|   IBIS model for TI am5k2e04 DSP
| -This IBIS model also supports am5k2e02
[IBIS Ver]   5.1
[Disclaimer]   Please be aware that in the absence of a written agreement
|   Texas Instruments(TI) assumes no liability for:
|   (1) The accuracy of the IBIS models provided to your company,
|   however, the IBIS model is compliant to industry standard
|   IQ Level 2a.  Refer to IBIS Quality Section below for
|   for full details.
|   (2) The proper functioning of these Models in your design
|   or for any resulting applications
|   (3) Infringement of patents, copyrights or intellectual
|   property rights resulting from your use of these
|   models.
|   z
|   TI provides IBIS Models as a service to our customers and
|   therefore reserves the right to limit distribution of the
|   Models.  The information is subject to change without notice.
[File Name]  am5k2e04_02_r1p2.ibs
[File Rev]   1.2
[Date]   28 August 2014
[Source]   Texas Instruments Incorporated
[Copyright]   Property of Texas Instruments Incorporated.
|   Unauthorized reproduction and/or distribution is strictly.
|   prohibited.
|   This product is protected under copyright law and trade
|   secret law as an unpublished work.
|   Created 2013,(C) Copyright 1999-2013,
|   Texas Instruments Incorporated., All Rights Reserved.
|   These commodities are under the U.S. Government
|   distribution license control. As such,they are not to be
|   re-exported without the prior approval of the U.S.
|   Department of Commerce.
[Notes]
   For SerDes simulations use Texas Instruments IBIS AMI models
   Some IV curves contain Non monotonic data points.
|   Model Generated by R.Lerner
|   **For SerDes simulations use Texas Instruments IBIS AMI models**
|   Revision History
|   GERNERAL COMMENT: All IBIS Quality Notes below reflect latest release
|   and version of IBIS File
|   Revision 1.2-- 28 August 2014
|   -Added naming for VMON pins.
|   Revision 1.1-- 25 August 2014
|   -Added the [Series Pin Mapping] to assign termination.
|   Revision 1.0-- 20 August 2014
|   -Updated the pin names to match the data manual.
|   Revision 0.9-- 25 October 2013
|   -Initial Release
|   Revision 0.8-- 25 October 2013
|   -Preliminary Release
|   Revision 0.1-- 20 October 2013
|   -Preliminary Model Generated
|   File passes ibischk 5.1.4 with 0 errors and 57 warnings
|   IBIS Quality Notes
|IQ
|IQ Component 66ak2e05: Overall Quality level 2a
|IQ
|IQ ibischk5 (5.1.4)
|IQ   -Parser for IBISCHK5 results
|IQ   - 20 instances where GND Clamp Minimum data is non-monotonic
|IQ   - 28 instances where GND Clamp Typical data is non-monotonic
|IQ   - 40 instances where Pulldown Maximum data is non-monotonic
|IQ   - 40 instances where Pulldown Typical data is non-monotonic
|IQ   - 40 instances where Pulldown Minimum data is non-monotonic
|IQ   - 32 instances where Pullup Maximum data is non-monotonic
|IQ   - 32 instances where Pullup Minimum data is non-monotonic
|IQ   - 32 instances where Pullup Typical data is non-monotonic
|IQ   - 12 instances where GND Clamp Maximum data is non-monotonic
|IQ   - 02 instances where POWER Clamp Maximum data is non-monotonic
|IQ   - 03 instances where ISSO_PU Typical data is non-monotonic
|IQ   - 06 instances where ISSO_PU Maximum data is non-monotonic
|IQ   - 06 instances where ISSO_PD Typical data is non-monotonic
|IQ   - 06 instances where ISSO_PD Minimum data is non-monotonic
|IQ   - 06 instances where ISSO_PD Maximum data is non-monotonic
|IQ   - 23 instances where Series_MOSFET Typical data is non-monotonic
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[Component] 66ak2e05
Si_location   Die
Timing_location Die
[Manufacturer] Texas Instruments
[Package Model] 66ak2eXX
[Package]
|Variable   Typ   Min   Max
|R_pkg   1.0013   0.15483   2.0653
|L_pkg   2.89689nH  0.94768nH   5.3815nH
|C_pkg   1.63791pF  0.87102pF   2.5609pF
R_pkg   1.7571   0.15793   3.744
L_pkg   7.0203nH  67.335pH   19.323nH
C_pkg   1.0304pF  0.61559pF   1.7804pF
[Pin] Signal_name model_name   | Buffer Name
A1   VSS   GND   | GND
A10   DDRDQS3P   DQS   | PDIFF_D3FF3_3L
A11   DDRD26   DQ   | PDDRIO_D3FP3_3L
A12   DDRCE0   ACC_OUT   | PDDRIO_D3FP3_3L
A13   DDRA10   ACC_OUT   | PDDRIO_D3FP3_3L
A14   RSV023   NC   | NC
A15   DDRCLKOUTN1   CLK_OUT   | PDDRIO_D3FP3_3L
A16   DDRCLKOUTP1   CLK_OUT   | PDDRIO_D3FP3_3L
A17   DDRA06   ACC_OUT   | PDDRIO_D3FP3_3L
A18   DDRA08   ACC_OUT   | PDDRIO_D3FP3_3L
A19   DDRCKE1   ACC_OUT   | PDDRIO_D3FP3_3L
A2   DVDD15   POWER   | POWER
A20   DDRCB06   DQ   | PDDRIO_D3FP3_3L
A21   DDRCB07   DQ   | PDDRIO_D3FP3_3L
A22   DDRDQS8N   DQS   | PDIFF_D3FF3_3L
A23   DDRCB00   DQ   | PDDRIO_D3FP3_3L
A24   DDRDQS4P   DQS   | PDIFF_D3FF3_3L
A25   DDRD39   DQ   | PDDRIO_D3FP3_3L
A26   DDRD45   DQ   | PDDRIO_D3FP3_3L
A27   DDRDQS5P   DQS   | PDIFF_D3FF3_3L
A28   DDRD49   DQ   | PDDRIO_D3FP3_3L
A29   DDRD48   DQ   | PDDRIO_D3FP3_3L
A3   DDRDQM0   DM   | PDDRIO_D3FP3_3L
A30   DDRDQS6P   DQS   | PDIFF_D3FF3_3L
A31   DDRDQM7   DM   | PDDRIO_D3FP3_3L
A32   DVDD15   POWER   | POWER
A33   VSS   GND   | GND
A4   DDRDQS1P   DQS   | PDIFF_D3FF3_3L
A5   DDRD08   DQ   | PDDRIO_D3FP3_3L
A6   DDRD09   DQ   | PDDRIO_D3FP3_3L
A7   DDRDQS2N   DQS   | PDIFF_D3FF3_3L
A8   DDRD22   DQ   | PDDRIO_D3FP3_3L
A9   DDRD31   DQ   | PDDRIO_D3FP3_3L
AA1   EMIFCE0   bc181540h   | bc181540edc50bghypbfbh
AA10   CVDD   POWER   | POWER
AA11   VSS   GND   | GND
AA12   CVDD1   POWER   | POWER
AA13   VSS   GND   | GND
AA14   CVDD1   POWER   | POWER
AA15   VSS   GND   | GND
AA16   CVDD   POWER   | POWER
AA17   VSS   GND   | GND
AA18   CVDD   POWER   | POWER
AA19   VSS   GND   | GND
AA2   EMIFBE0   bc181540h   | bc181540edc50bghypbfbh
AA20   CVDD   POWER   | POWER
AA21   VSS   GND   | GND
AA22   CVDD   POWER   | POWER
AA23   VSS   GND   | GND
AA24   CVDD1   POWER   | POWER
AA25   VSS   GND   | GND
AA26   CVDD   POWER   | POWER
AA27   VSS   GND   | GND
AA28   DVDD18   POWER   | POWER
AA29   GPIO01   bc181540h   | bc181540edc50bghypbfbh
AA3   DVDD18   POWER   | POWER
AA30   GPIO13   bc181540h   | bc181540edc50bghypbfbh
AA31   DVDD18   POWER   | POWER
AA32   VSS   GND   | GND
AA33   GPIO16   bc181540h   | bc181540edc50bghypbfbh
AA4   VSS   GND   | GND
AA5   EMU15   bc181540h   | bc181540edc50bghypbfbh
AA6   EMU01   bc181540h   | bc181540edc50bghypbfbh
AA7   VSS   GND   | GND
AA8   DVDD18   POWER   | POWER
AA9   VSS   GND   | GND
AB1   USB0DRVVBUS   bc181540h   | bc181540edc50bghypbfbh
AB10   VSS   GND   | GND
AB11   CVDD   POWER   | POWER
AB12   VSS   GND   | GND
AB13   CVDD   POWER   | POWER
AB14   VSS   GND   | GND
AB15   CVDD   POWER   | POWER
AB16   VSS   GND   | GND
AB17   CVDD   POWER   | POWER
AB18   VSS   GND   | GND
AB19   CVDD   POWER   | POWER
AB2   EMU16   bc181540h   | bc181540edc50bghypbfbh
AB20   VSS   GND   | GND
AB21   CVDD   POWER   | POWER
AB22   VSS   GND   | GND
AB23   CVDD1   POWER   | POWER
AB24   VSS   GND   | GND
AB25   CVDD   POWER   | POWER
AB26   VSS   GND   | GND
AB27   DVDD18   POWER   | POWER
AB28   VSS   GND   | GND
AB29   GPIO10   bc181540h   | bc181540edc50bghypbfbh
AB3   EMU14   bc181540h   | bc181540edc50bghypbfbh
AB30   GPIO25   bc181540h   | bc181540edc50bghypbfbh
AB31   GPIO19   bc181540h   | bc181540edc50bghypbfbh
AB32   GPIO17   bc181540h   | bc181540edc50bghypbfbh
AB33   GPIO18   bc181540h   | bc181540edc50bghypbfbh
AB4   EMU08   bc181540h   | bc181540edc50bghypbfbh
AB5   EMU06   bc181540h   | bc181540edc50bghypbfbh
AB6   HYPLNK0TXPMCLK  bc181540h   | bc181540edc50bghypbfbh
AB7   DVDD18   POWER   | POWER
AB8   VSS   GND   | GND
AB9   CVDD   POWER   | POWER
AC1   USB1DRVVBUS   POWER   | POWER
AC10   CVDD   POWER   | POWER
AC11   VSS   GND   | GND
AC12   CVDD   POWER   | POWER
AC13   VSS   GND   | GND
AC14   CVDD   POWER   | POWER
AC15   VSS   GND   | GND
AC16   CVDD   POWER   | POWER
AC17   VSS   GND   | GND
AC18   CVDD   POWER   | POWER
AC19   VSS   GND   | GND
AC2   EMU13   bc181540h   | bc181540edc50bghypbfbh
AC20   CVDD   POWER   | POWER
AC21   VSS   GND   | GND
AC22   CVDD   POWER   | POWER
AC23   VSS   GND   | GND
AC24   CVDD   POWER   | POWER
AC25   VSS   GND   | GND
AC26   CVDD   POWER   | POWER
AC27   VSS   GND   | GND
AC28   DVDD18   POWER   | POWER
AC29   GPIO20   bc181540h   | bc181540edc50bghypbfbh
AC3   EMU07   bc181540h   | bc181540edc50bghypbfbh
AC30   GPIO26   bc181540h   | bc181540edc50bghypbfbh
AC31   GPIO23   bc181540h   | bc181540edc50bghypbfbh
AC32   GPIO24   bc181540h   | bc181540edc50bghypbfbh
AC33   GPIO21   bc181540h   | bc181540edc50bghypbfbh
AC4   EMU02   bc181540h   | bc181540edc50bghypbfbh
AC5   EMU00   bc181540h   | bc181540edc50bghypbfbh
AC6   HYPLNK0TXFLCLK  bc181540h   | bc181540edc50bghypbfbh
AC7   VSS   GND   | GND
AC8   DVDD18   POWER   | POWER
AC9   VSS   GND   | GND
AD1   HYPLNK0RXPMDAT  bc181540h   | bc181540edc50bghypbfbh
AD10   VSS   GND   | GND
AD11   CVDD   POWER   | POWER
AD12   VSS   GND   | GND
AD13   CVDD   POWER   | POWER
AD14   VSS   GND   | GND
AD15   CVDD   POWER   | POWER
AD16   VSS   GND   | GND
AD17   CVDD   POWER   | POWER
AD18   VSS   GND   | GND
AD19   CVDD   POWER   | POWER
AD2   EMU12   bc181540h   | bc181540edc50bghypbfbh
AD20   VSS   GND   | GND
AD21   CVDD   POWER   | POWER
AD22   VSS   GND   | GND
AD23   VNWA3   POWER   | POWER
AD24   VSS   GND   | GND
AD25   CVDD   POWER   | POWER
AD26   VSS   GND   | GND
AD27   DVDD18   POWER   | POWER
AD28   VSS   GND   | GND
AD29   GPIO22   bc181540h   | bc181540edc50bghypbfbh
AD3   EMU05   bc181540h   | bc181540edc50bghypbfbh
AD30   GPIO31   bc181540h   | bc181540edc50bghypbfbh
AD31   GPIO29   bc181540h   | bc181540edc50bghypbfbh
AD32   GPIO27   bc181540h   | bc181540edc50bghypbfbh
AD33   GPIO28   bc181540h   | bc181540edc50bghypbfbh
AD4   DVDD18   POWER   | POWER
AD5   VSS   GND   | GND
AD6   EMU04   bc181540h   | bc181540edc50bghypbfbh
AD7   AVDDA3   POWER   | POWER
AD8   VSS   GND   | GND
AD9   VNWA4   POWER   | POWER
AE1   HYPLNK0RXPMCLK  bc181540h   | bc181540edc50bghypbfbh
AE10   VDDALV   POWER   | POWER
AE11   VSS   GND   | GND
AE12   VDDALV   POWER   | POWER
AE13   VSS   GND   | GND
AE14   VDDALV   POWER   | POWER
AE15   VSS   GND   | GND
AE16   VDDALV   POWER   | POWER
AE17   VSS   GND   | GND
AE18   VDDALV   POWER   | POWER
AE19   VSS   GND   | GND
AE2   RSV002   NC   | NC
AE20   VDDALV   POWER   | POWER
AE21   VSS   GND   | GND
AE22   VDDALV   POWER   | POWER
AE23   VSS   GND   | GND
AE24   VDDALV   POWER   | POWER
AE25   VSS   GND   | GND
AE26   DVDD18   POWER   | POWER
AE27   VSS   GND   | GND
AE28   DVDD18   POWER   | POWER
AE29   RESET   ic1815ghypbfbh  | ic1815ghypbfbh
AE3   HYPLNK0RXFLDAT  bc181540h   | bc181540edc50bghypbfbh
AE30   RSV030   bc181540h   | bc181540edc50bghypbfbh
AE31   DVDD18   POWER   | POWER
AE32   VSS   GND   | GND
AE33   GPIO30   bc181540h   | bc181540edc50bghypbfbh
AE4   SYSCLKOUT   bc181540h   | bc181540edc50bghypbfbh
AE5   TSSYNCEVT   bc181540h   | bc181540edc50bghypbfbh
AE6   EMU03   bc181540h   | bc181540edc50bghypbfbh
AE7   XFIMDIO   bc181540h   | bc181540edc50bghypbfbh
AE8   DVDD18   POWER   | POWER
AE9   VSS   GND   | GND
AF1   CORECLKP   iclkrx0p9gh   | iclkrx0p9gh
AF10   VSS   GND   | GND
AF11   VDDALV   POWER   | POWER
AF12   VSS   GND   | GND
AF13   VDDALV   POWER   | POWER
AF14   VSS   GND   | GND
AF15   VDDALV   POWER   | POWER
AF16   VSS   GND   | GND
AF17   VDDALV   POWER   | POWER
AF18   VSS   GND   | GND
AF19   VDDALV   POWER   | POWER
AF2   RSV003   NC   | NC
AF20   VSS   GND   | GND
AF21   VDDALV   POWER   | POWER
AF22   VSS   GND   | GND
AF23   VDDALV   POWER   | POWER
AF24   VSS   GND   | GND
AF25   VDDALV   POWER   | POWER
AF26   VSS   GND   | GND
AF27   DVDD18   POWER   | POWER
AF28   VSS   GND   | GND
AF29   TDO   bc181540h   | bc181540edc50bghypbfbh
AF3   EMU10   bc181540h   | bc181540edc50bghypbfbh
AF30   HOUT   bc181540h   | bc181540edc50bghypbfbh
AF31   BOOTCOMPLETE   bc181540h   | bc181540edc50bghypbfbh
AF32   RESETFULL   bc181540h   | bc181540edc50bghypbfbh
AF33   RSV029   bc181540h   | bc181540edc50bghypbfbh
AF4   TSCOMPOUT   bc181540h   | bc181540edc50bghypbfbh
AF5   HYPLNK0TXPMDAT  bc181540h   | bc181540edc50bghypbfbh
AF6   XFIMDCLK   bc181540h   | bc181540edc50bghypbfbh
AF7   AVDDA1   POWER   | POWER
AF8   VSS   GND   | GND
AF9   VDDALV   POWER   | POWER
AG1   CORECLKN   iclkrx0p9gh   | iclkrx0p9gh
AG10   XFIREFRES0   NC   | NC
AG11   VSS   GND   | GND
AG12   RSV017   NC   | NC
AG13   VSS   GND   | GND
AG14   PCIE0REFRES   NC   | NC
AG15   VSS   GND   | GND
AG16   VDDALV   POWER   | POWER
AG17   VSS   GND   | GND
AG18   VDDALV   POWER   | POWER
AG19   VSS   GND   | GND
AG2   TSRXCLKOUT1P   olvds18gh | olvds18gh
AG20   VDDALV   POWER   | POWER
AG21   VSS   GND   | GND
AG22   VDDALV   POWER   | POWER
AG23   VSS   GND   | GND
AG24   VDDALV   POWER   | POWER
AG25   VSS   GND   | GND
AG26   DVDD18   POWER   | POWER
AG27   VSS   GND   | GND
AG28   SDA0   bi2c1815gfzhsh  | bi2c1815gfzhsh
AG29   SDA2   bi2c1815gfzhsh  | bi2c1815gfzhsh
AG3   TSPUSHEVT0   bc181540h   | bc181540edc50bghypbfbh
AG30   SCL0   bi2c1815gfzhsh  | bi2c1815gfzhsh
AG31   TDI   ic1815ghypbfbh  | ic1815ghypbfbh
AG32   TRST   ic1815ghypbfbh  | ic1815ghypbfbh
AG33   RSV028   bc181540h   | bc181540edc50bghypbfbh
AG4   EMU11   bc181540h   | bc181540edc50bghypbfbh
AG5   RSV008   NC   | NC
AG6   NETCPCLKSEL   ic1815ghypbfbh  | ic1815ghypbfbh
AG7   VSS   GND   | GND
AG8   RSV015   NC   | NC
AG9   VSS   GND   | GND
AH1   TSRXCLKOUT1N   olvds18gh   | olvds18gh
AH10   VSS   GND   | GND
AH11   VDDAHV   POWER   | POWER
AH12   VSS   GND   | GND
AH13   VDDAHV   POWER   | POWER
AH14   VSS   GND   | GND
AH15   VDDAHV   POWER   | POWER
AH16   VSS   GND   | GND
AH17   VDDAHV   POWER   | POWER
AH18   VSS   GND   | GND
AH19   VDDAHV   POWER   | POWER
AH2   EMU18   bc181540h   | bc181540edc50bghypbfbh
AH20   VSS   GND   | GND
AH21   VDDAHV   POWER   | POWER
AH22   VSS   GND   | GND
AH23   VDDAHV   POWER   | POWER
AH24   VSS   GND   | GND
AH25   VDDAHV   POWER   | POWER
AH26   VSS   GND   | GND
AH27   DVDD18   POWER   | POWER
AH28   VSS   GND   | GND
AH29   RESETSTAT   bc181540h   | bc181540edc50bghypbfbh
AH3   EMU09   bc181540h   | bc181540edc50bghypbfbh
AH30   SCL1   bi2c1815gfzhsh  | bi2c1815gfzhsh
AH31   SCL2   bi2c1815gfzhsh  | bi2c1815gfzhsh
AH32   TMS   ic1815ghypbfbh  | ic1815ghypbfbh
AH33   POR   ihhv181512ghyh  | ihhv181512ghyh
AH4   HYPLNK0TXFLDAT  bc181540h   | bc181540edc50bghypbfbh
AH5   MDIO0   bc181540h   | bc181540edc50bghypbfbh
AH6   MDCLK0   bc181540h   | bc181540edc50bghypbfbh
AH7   XFIREFRES1   NC   | NC
AH8   VSS   GND   | GND
AH9   RSV020   NC   | NC
AJ1   TSRXCLKOUT0P   olvds18gh   | olvds18gh
AJ10   PCIE1REFRES   NC   | NC
AJ11   XFICLKP   NC   | NC
AJ12   XFICLKN   NC   | NC
AJ13   VSS   GND   | GND
AJ14   PCIE1CLKP   NC   | SERDES
AJ15   PCIE1CLKN   NC   | SERDES
AJ16   VSS   GND   | GND
AJ17   PCIE0CLKP   NC   | SERDES
AJ18   PCIE0CLKN   NC   | SERDES
AJ19   VSS   GND   | GND
AJ2   TSRXCLKOUT0N   olvds18gh   | olvds18gh
AJ20   RSV016   NC   | NC
AJ21   VSS   GND   | GND
AJ22   SGMII01REFRES   NC   | NC
AJ23   VSS   GND   | GND
AJ24   SGMII0CLKP   iclkrx0p9gh   | iclkrx0p9gv
AJ25   SGMII0CLKN   iclkrx0p9gh   | iclkrx0p9gv
AJ26   RSV019   NC   | NC
AJ27   SGMII00REFRES   NC   | NC
AJ28   RSV018   NC   | NC
AJ29   VSS   GND   | GND
AJ3   HYPLNK0RXFLCLK  bc181540h   | bc181540edc50bghypbfbh
AJ30   DVDD18   POWER   | POWER
AJ31   TSIP0FSA   bc181540h   | bc181540edc50bghypbfbh
AJ32   SDA1   bi2c1815gfzhsh  | bi2c1815gfzhsh
AJ33   TCK   ic1815ghypbfbh  | ic1815ghypbfbh
AJ4   VSS   GND   | GND
AJ5   HYPLNK0REFRES   NC   | NC
AJ6   VSS   GND   | GND
AJ7   HYPLNK0CLKP   NC   | SERDES
AJ8   HYPLNK0CLKN   NC   | SERDES
AJ9   VSS   GND   | GND
AK1   TSREFCLKN   NC   | ilvds18gh
AK10   XFITXP1   NC   | SERDES
AK11   XFITXN1   NC   | SERDES
AK12   VSS   GND   | GND
AK13   PCIE1TXP1   NC   | SERDES
AK14   PCIE1TXN1   NC   | SERDES
AK15   VSS   GND   | GND
AK16   PCIE0TXP1   NC   | SERDES
AK17   PCIE0TXN1   NC   | SERDES
AK18   VSS   GND   | GND
AK19   SGMII0TXP7   NC   | SERDES
AK2   TSREFCLKP   NC   | ilvds18gh
AK20   SGMII0TXN7   NC   | SERDES
AK21   VSS   GND   | GND
AK22   SGMII0TXP5   NC   | SERDES
AK23   SGMII0TXN5   NC   | SERDES
AK24   VSS   GND   | GND
AK25   SGMII0TXP3   NC   | SERDES
AK26   SGMII0TXN3   NC   | SERDES
AK27   VSS   GND   | GND
AK28   SGMII0TXP1   NC   | SERDES
AK29   SGMII0TXN1   NC   | SERDES
AK3   VSS   GND   | GND
AK30   VSS   GND   | GND
AK31   TSIP0CLKA   bc181540h   | bc181540edc50bghypbfbh
AK32   TSIP0FSB   bc181540h   | bc181540edc50bghypbfbh
AK33   TSIP0CLKB   bc181540h   | bc181540edc50bghypbfbh
AK4   HYPLNK0TXP3   NC   | SERDES
AK5   HYPLNK0TXN3   NC   | SERDES
AK6   VSS   GND   | GND
AK7   HYPLNK0TXP1   NC   | SERDES
AK8   HYPLNK0TXN1   NC   | SERDES
AK9   VSS   GND   | GND
AL1   TSPUSHEVT1   bc181540h   | bc181540edc50bghypbfbh
AL10   VSS   GND   | GND
AL11   XFITXP0   NC   | SERDES
AL12   XFITXN0   NC   | SERDES
AL13   VSS   GND   | GND
AL14   PCIE1TXP0   NC   | SERDES
AL15   PCIE1TXN0   NC   | SERDES
AL16   VSS   GND   | GND
AL17   PCIE0TXP0   NC   | SERDES
AL18   PCIE0TXN0   NC   | SERDES
AL19   VSS   GND   | GND
AL2   RSV007   NC   | NC
AL20   SGMII0TXP6   NC   | SERDES
AL21   SGMII0TXN6   NC   | SERDES
AL22   VSS   GND   | GND
AL23   SGMII0TXP4   NC   | SERDES
AL24   SGMII0TXN4   NC   | SERDES
AL25   VSS   GND   | GND
AL26   SGMII0TXP2   NC   | SERDES
AL27   SGMII0TXN2   NC   | SERDES
AL28   VSS   GND   | GND
AL29   SGMII0TXP0   NC   | SERDES
AL3   RSV006   NC   | NC
AL30   SGMII0TXN0   NC   | SERDES
AL31   VSS   GND   | GND
AL32   TSIP0TX0   bc181540h   | bc181540edc50bghypbfbh
AL33   TSIP0TR1   bc181540h   | bc181540edc50bghypbfbh
AL4   VSS   GND   | GND
AL5   HYPLNK0TXP2   NC   | SERDES
AL6   HYPLNK0TXN2   NC   | SERDES
AL7   VSS   GND   | GND
AL8   HYPLNK0TXP0   NC   | SERDES
AL9   HYPLNK0TXN0   NC   | SERDES
AM1   VSS   GND   | GND
AM10   XFIRXN1   NC   | SERDES
AM11   XFIRXP1   NC   | SERDES
AM12   VSS   GND   | GND
AM13   PCIE1RXN1   NC   | SERDES
AM14   PCIE1RXP1   NC   | SERDES
AM15   VSS   GND   | GND
AM16   PCIE0RXN1   NC   | SERDES
AM17   PCIE0RXP1   NC   | SERDES
AM18   VSS   GND   | GND
AM19   SGMII0RXN7   NC   | SERDES
AM2   NETCPCLKP   iclkrx0p9gh   | iclkrx0p9gh
AM20   SGMII0RXP7   NC   | SERDES
AM21   VSS   GND   | GND
AM22   SGMII0RXN5   NC   | SERDES
AM23   SGMII0RXP5   NC   | SERDES
AM24   VSS   GND   | GND
AM25   SGMII0RXN3   NC   | SERDES
AM26   SGMII0RXP3   NC   | SERDES
AM27   VSS   GND   | GND
AM28   SGMII0RXN1   NC   | SERDES
AM29   SGMII0RXP1   NC   | SERDES
AM3   VSS   GND   | GND
AM30   VSS   GND   | GND
AM31   TSIP0TR0   bc181540h   | bc181540edc50bghypbfbh
AM32   TSIP0TX1   bc181540h   | bc181540edc50bghypbfbh
AM33   DVDD18   POWER   | POWER
AM4   HYPLNK0RXN3   NC   | SERDES
AM5   HYPLNK0RXP3   NC   | SERDES
AM6   VSS   GND   | GND
AM7   HYPLNK0RXN1   NC   | SERDES
AM8   HYPLNK0RXP1   NC   | SERDES
AM9   VSS   GND   | GND
AN1   VSS   GND   | GND
AN10   VSS   GND   | GND
AN11   XFIRXN0   NC   | SERDES
AN12   XFIRXP0   NC   | SERDES
AN13   VSS   GND   | GND
AN14   PCIE1RXN0   NC   | SERDES
AN15   PCIE1RXP0   NC   | SERDES
AN16   VSS   GND   | GND
AN17   PCIE0RXN0   NC   | SERDES
AN18   PCIE0RXP0   NC   | SERDES
AN19   VSS   GND   | GND
AN2   VSS   GND   | GND
AN20   SGMII0RXN6   NC   | SERDES
AN21   SGMII0RXP6   NC   | SERDES
AN22   VSS   GND   | GND
AN23   SGMII0RXN4   NC   | SERDES
AN24   SGMII0RXP4   NC   | SERDES
AN25   VSS   GND   | GND
AN26   SGMII0RXN2   NC   | SERDES
AN27   SGMII0RXP2   NC   | SERDES
AN28   VSS   GND   | GND
AN29   SGMII0RXN0   NC   | SERDES
AN3   NETCPCLKN   iclkrx0p9gh   | iclkrx0p9gh
AN30   SGMII0RXP0   NC   | SERDES
AN31   VSS   GND   | GND
AN32   DVDD18   POWER   | POWER
AN33   VSS   GND   | GND
AN4   VSS   GND   | GND
AN5   HYPLNK0RXN2   NC   | SERDES
AN6   HYPLNK0RXP2   NC   | SERDES
AN7   VSS   GND   | GND
AN8   HYPLNK0RXN0   NC   | SERDES
AN9   HYPLNK0RXP0   NC   | SERDES
B1   DVDD15   POWER   | POWER
B10   DDRDQS3N   DQS   | PDIFF_D3FF3_3L
B11   DDRD25   DQ   | PDDRIO_D3FP3_3L
B12   DDRCAS   ACC_OUT   | PDDRIO_D3FP3_3L
B13   DDRRAS   ACC_OUT   | PDDRIO_D3FP3_3L
B14   DDRCLKOUTN0   CLK_OUT   | PDDRIO_D3FP3_3L
B15   DDRCLKOUTP0   CLK_OUT   | PDDRIO_D3FP3_3L
B16   DDRA02   ACC_OUT   | PDDRIO_D3FP3_3L
B17   DDRA09   ACC_OUT   | PDDRIO_D3FP3_3L
B18   DDRBA2   ACC_OUT   | PDDRIO_D3FP3_3L
B19   RSV021   NC   | NC
B2   DDRD07   DQ   | PDDRIO_D3FP3_3L
B20   DDRDQM8   DM   | PDDRIO_D3FP3_3L
B21   DDRCB05   DQ   | PDDRIO_D3FP3_3L
B22   DDRDQS8P   DQS   | PDIFF_D3FF3_3L
B23   DDRD32   DQ   | PDDRIO_D3FP3_3L
B24   DDRDQS4N   DQS   | PDIFF_D3FF3_3L
B25   DDRD38   DQ   | PDDRIO_D3FP3_3L
B26   DDRD46   DQ   | PDDRIO_D3FP3_3L
B27   DDRDQS5N   DQS   | PDIFF_D3FF3_3L
B28   DDRD44   DQ   | PDDRIO_D3FP3_3L
B29   DDRD52   DQ   | PDDRIO_D3FP3_3L
B3   DDRD15   DQ   | PDDRIO_D3FP3_3L
B30   DDRDQS6N   DQS   | PDIFF_D3FF3_3L
B31   DDRD50   DQ   | PDDRIO_D3FP3_3L
B32   DDRD63   DQ   | PDDRIO_D3FP3_3L
B33   DVDD15   POWER   | POWER
B4   DDRDQS1N   DQS   | PDIFF_D3FF3_3L
B5   DDRD10   DQ   | PDDRIO_D3FP3_3L
B6   DDRD19   DQ   | PDDRIO_D3FP3_3L
B7   DDRDQS2P   DQS   | PDIFF_D3FF3_3L
B8   DDRD23   DQ   | PDDRIO_D3FP3_3L
B9   DDRD29   DQ   | PDDRIO_D3FP3_3L
C1   DDRDQS0P   DQS   | PDIFF_D3FF3_3L
C10   DDRD27   DQ   | PDDRIO_D3FP3_3L
C11   DVDD15   POWER   | POWER
C12   DDRCE1   ACC_OUT   | PDDRIO_D3FP3_3L
C13   DDRBA1   ACC_OUT   | PDDRIO_D3FP3_3L
C14   VSS   GND   | GND
C15   DDRA01   ACC_OUT   | PDDRIO_D3FP3_3L
C16   DDRA03   ACC_OUT   | PDDRIO_D3FP3_3L
C17   DVDD15   POWER   | POWER
C18   DDRA14   ACC_OUT   | PDDRIO_D3FP3_3L
C19   VSS   GND   | GND
C2   DDRDQS0N   DQS   | PDIFF_D3FF3_3L
C20   DDRCKE0   ACC_OUT   | PDDRIO_D3FP3_3L
C21   DVDD15   POWER   | POWER
C22   DDRCB04   DQ   | PDDRIO_D3FP3_3L
C23   VSS   GND   | GND
C24   DDRD35   DQ   | PDDRIO_D3FP3_3L
C25   DVDD15   POWER   | POWER
C26   DDRD47   DQ   | PDDRIO_D3FP3_3L
C27   VSS   GND   | GND
C28   DDRD42   DQ   | PDDRIO_D3FP3_3L
C29   VSS   GND   | GND
C3   DVDD15   POWER   | POWER
C30   DDRD53   DQ   | PDDRIO_D3FP3_3L
C31   DVDD15   POWER   | POWER
C32   DDRD61   DQ   | PDDRIO_D3FP3_3L
C33   DDRDQS7P   DQS   | PDIFF_D3FF3_3L
C4   DDRD12   DQ   | PDDRIO_D3FP3_3L
C5   VSS   GND   | GND
C6   DDRD20   DQ   | PDDRIO_D3FP3_3L
C7   DVDD15   POWER   | POWER
C8   DDRD21   DQ   | PDDRIO_D3FP3_3L
C9   VSS   GND   | GND
D1   DDRD01   DQ   | PDDRIO_D3FP3_3L
D10   DDRD28   DQ   | PDDRIO_D3FP3_3L
D11   VSS   GND   | GND
D12   DDRODT0   ACC_OUT   | PDDRIO_D3FP3_3L
D13   DDRBA0   ACC_OUT   | PDDRIO_D3FP3_3L
D14   DVDD15   POWER   | POWER
D15   DDRA00   ACC_OUT   | PDDRIO_D3FP3_3L
D16   DDRA04   ACC_OUT   | PDDRIO_D3FP3_3L
D17   VSS   GND   | GND
D18   DDRA11   ACC_OUT   | PDDRIO_D3FP3_3L
D19   DVDD15   POWER   | POWER
D2   DDRD05   DQ   | PDDRIO_D3FP3_3L
D20   DDRRESET   ACC_OUT   | PDDRIO_D3FP3_3L
D21   VSS   GND   | GND
D22   DDRCB01   DQ   | PDDRIO_D3FP3_3L
D23   DVDD15   POWER   | POWER
D24   DDRD34   DQ   | PDDRIO_D3FP3_3L
D25   VSS   GND   | GND
D26   DDRDQM5   DM   | PDDRIO_D3FP3_3L
D27   DVDD15   POWER   | POWER
D28   DDRD41   DQ   | PDDRIO_D3FP3_3L
D29   DVDD15   POWER   | POWER
D3   VSS   GND   | GND
D30   DDRD55   DQ   | PDDRIO_D3FP3_3L
D31   VSS   GND   | GND
D32   DDRD62   DQ   | PDDRIO_D3FP3_3L
D33   DDRDQS7N   DQS   | PDIFF_D3FF3_3L
D4   DDRD13   DQ   | PDDRIO_D3FP3_3L
D5   DVDD15   POWER   | POWER
D6   DDRD16   DQ   | PDDRIO_D3FP3_3L
D7   VSS   GND   | GND
D8   DDRDQM2   DM   | PDDRIO_D3FP3_3L
D9   DVDD15   POWER   | POWER
E1   DDRD03   DQ   | PDDRIO_D3FP3_3L
E10   DDRD24   DQ   | PDDRIO_D3FP3_3L
E11   DDRODT1   ACC_OUT   | PDDRIO_D3FP3_3L
E12   DDRA13   ACC_OUT   | PDDRIO_D3FP3_3L
E13   DDRWE   ACC_OUT   | PDDRIO_D3FP3_3L
E14   AVDDA7   POWER   | POWER
E15   DDRRZQ0   NC   | D3F_PZQ_NS
E16   DDRA05   ACC_OUT   | PDDRIO_D3FP3_3L
E17   DDRA07   ACC_OUT   | PDDRIO_D3FP3_3L
E18   DDRA12   ACC_OUT   | PDDRIO_D3FP3_3L
E19   DDRA15   ACC_OUT   | PDDRIO_D3FP3_3L
E2   DDRD00   DQ   | PDDRIO_D3FP3_3L
E20   RSV022   NC   | NC
E21   DDRCB03   DQ   | PDDRIO_D3FP3_3L
E22   DDRCB02   DQ   | PDDRIO_D3FP3_3L
E23   DDRD33   DQ   | PDDRIO_D3FP3_3L
E24   DDRD36   DQ   | PDDRIO_D3FP3_3L
E25   DDRD37   DQ   | PDDRIO_D3FP3_3L
E26   DDRDQM4   DM   | PDDRIO_D3FP3_3L
E27   DDRD43   DQ   | PDDRIO_D3FP3_3L
E28   DDRD40   DQ   | PDDRIO_D3FP3_3L
E29   DDRD51   DQ   | PDDRIO_D3FP3_3L
E3   DDRDQM1   DM   | PDDRIO_D3FP3_3L
E30   DDRD54   DQ   | PDDRIO_D3FP3_3L
E31   DDRDQM6   DM   | PDDRIO_D3FP3_3L
E32   DDRD59   DQ   | PDDRIO_D3FP3_3L
E33   DDRD60   DQ   | PDDRIO_D3FP3_3L
E4   DDRD14   DQ   | PDDRIO_D3FP3_3L
E5   DDRD11   DQ   | PDDRIO_D3FP3_3L
E6   DDRD17   DQ   | PDDRIO_D3FP3_3L
E7   DDRD18   DQ   | PDDRIO_D3FP3_3L
E8   DDRDQM3   DM   | PDDRIO_D3FP3_3L
E9   DDRD30   DQ   | PDDRIO_D3FP3_3L
F1   DDRD04   DQ   | PDDRIO_D3FP3_3L
F10   VSS   GND   | GND
F11   DVDD15   POWER   | POWER
F12   VSS   GND   | GND
F13   DVDD15   POWER   | POWER
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|********************  DIFF PIN  *******************************
[Diff_pin]   inv_pin vdiff tdelay_typ   tdelay_min  tdelay_max
AG1   AF1   200mV   NA   NA   NA   || CORECLKN & CORECLKP
B14   B15   200mV   NA   NA   NA   || DDRCLKOUTN0 & DDRCLKOUTP0
A16   A15   200mV   NA   NA   NA   || DDRCLKOUTP1 & DDRCLKOUTN1
C2   C1   200mV   NA   NA   NA   || DDRDQS0N & DDRDQS0P
B4   A4   200mV   NA   NA   NA   || DDRDQS1N & DDRDQS1P
A7   B7   200mV   NA   NA   NA   || DDRDQS2N & DDRDQS2P
B10   A10   200mV   NA   NA   NA   || DDRDQS3N & DDRDQS3P
B24   A24   200mV   NA   NA   NA   || DDRDQS4N & DDRDQS4P
B27   A27   200mV   NA   NA   NA   || DDRDQS5N & DDRDQS5P
B30   A30   200mV   NA   NA   NA   || DDRDQS6N & DDRDQS6P
D33   C33   200mV   NA   NA   NA   || DDRDQS7N & DDRDQS7P
A22   B22   200mV   NA   NA   NA   || DDRDQS8N & DDRDQS8P
AN8   AN9   50mV   NA   NA   NA   || HYPLNK0RXN0 & HYPLNK0RXP0
AM7   AM8   50mV   NA   NA   NA   || HYPLNK0RXN1 & HYPLNK0RXP1
AN5   AN6   50mV   NA   NA   NA   || HYPLNK0RXN2 & HYPLNK0RXP2
AM4   AM5   50mV   NA   NA   NA   || HYPLNK0RXN3 & HYPLNK0RXP3
AL9   AL8   50mV   NA   NA   NA   || HYPLNK0TXN0 & HYPLNK0TXP0
AK8   AK7   50mV   NA   NA   NA   || HYPLNK0TXN1 & HYPLNK0TXP1
AL6   AL5   50mV   NA   NA   NA   || HYPLNK0TXN2 & HYPLNK0TXP2
AK5   AK4   50mV   NA   NA   NA   || HYPLNK0TXN3 & HYPLNK0TXP3
AM2   AN3   200mV   NA   NA   NA   || NETCPCLKP & NETCPCLKN
AJ18   AJ17   50mV   NA   NA   NA   || PCIE0CLKN & PCIE0CLKP
AN17   AN18   50mV   NA   NA   NA   || PCIE0RXN0 & PCIE0RXP0
AM16   AM17   50mV   NA   NA   NA   || PCIE0RXN1 & PCIE0RXP1
AL18   AL17   50mV   NA   NA   NA   || PCIE0TXN0 & PCIE0TXP0
AK17   AK16   50mV   NA   NA   NA   || PCIE0TXN1 & PCIE0TXP1
AJ15   AJ14   50mV   NA   NA   NA   || PCIE1CLKN & PCIE1CLKP
AN14   AN15   50mV   NA   NA   NA   || PCIE1RXN0 & PCIE1RXP0
AM13   AM14   50mV   NA   NA   NA   || PCIE1RXN1 & PCIE1RXP1
AL15   AL14   50mV   NA   NA   NA   || PCIE1TXN0 & PCIE1TXP0
AK14   AK13   50mV   NA   NA   NA   || PCIE1TXN1 & PCIE1TXP1
AJ25   AJ24   50mV   NA   NA   NA   || SGMII0CLKN & SGMII0CLKP
AN29   AN30   50mV   NA   NA   NA   || SGMII0RXN0 & SGMII0RXP0
AM28   AM29   50mV   NA   NA   NA   || SGMII0RXN1 & SGMII0RXP1
AN26   AN27   50mV   NA   NA   NA   || SGMII0RXN2 & SGMII0RXP2
AM25   AM26   50mV   NA   NA   NA   || SGMII0RXN3 & SGMII0RXP3
AN23   AN24   50mV   NA   NA   NA   || SGMII0RXN4 & SGMII0RXP4
AM22   AM23   50mV   NA   NA   NA   || SGMII0RXN5 & SGMII0RXP5
AN20   AN21   50mV   NA   NA   NA   || SGMII0RXN6 & SGMII0RXP6
AM19   AM20   50mV   NA   NA   NA   || SGMII0RXN7 & SGMII0RXP7
AL30   AL29   50mV   NA   NA   NA   || SGMII0TXN0 & SGMII0TXP0
AK29   AK28   50mV   NA   NA   NA   || SGMII0TXN1 & SGMII0TXP1
AL27   AL26   50mV   NA   NA   NA   || SGMII0TXN2 & SGMII0TXP2
AK26   AK25   50mV   NA   NA   NA   || SGMII0TXN3 & SGMII0TXP3
AL24   AL23   50mV   NA   NA   NA   || SGMII0TXN4 & SGMII0TXP4
AK23   AK22   50mV   NA   NA   NA   || SGMII0TXN5 & SGMII0TXP5
AL21   AL20   50mV   NA   NA   NA   || SGMII0TXN6 & SGMII0TXP6
AK20   AK19   50mV   NA   NA   NA   || SGMII0TXN7 & SGMII0TXP7
AK1   AK2   50mV   NA   NA   NA   || TSREFCLKN & TSREFCLKP
AJ2   AJ1   50mV   NA   NA   NA   || TSRXCLKOUT0N & TSRXCLKOUT0P
AH1   AG2   50mV   NA   NA   NA   || TSRXCLKOUT1N & TSRXCLKOUT1P
W3   V3   NA   NA   NA   NA   || USB0DM & USB0DP
T1   U1   NA   NA   NA   NA   || USB0RX0M & USB0RX0P
U2   V2   NA   NA   NA   NA   || USB0TX0M & USB0TX0P
P4   R4   NA   NA   NA   NA   || USB1DM & USB1DP
N1   P1   NA   NA   NA   NA   || USB1RX0M & USB1RX0P
R2   P2   NA   NA   NA   NA   || USB1TX0M & USB1TX0P
T4   U4   NA   NA   NA   NA   || USBCLKM & USBCLKP
AJ12   AJ11   50mV   NA   NA   NA   || XFICLKN & XFICLKP
AN11   AN12   50mV   NA   NA   NA   || XFIRXN0 & XFIPXN0
AM10   AM11   50mV   NA   NA   NA   || XFIRXN1 & XFIRXN1
AL12   AL11   50mV   NA   NA   NA   || XFITXN0 & XFITXP0
AK11   AK10   50mV   NA   NA   NA   || XFITXN1 & XFITXP1
[Series Pin Mapping]   pin_2   model_name
G4   G3   s_iclkrx0p9gh   || DDRCLKN/P
AJ24   AJ25   s_iclkrx0p9gv   || SGMII0CLKN/P
U4   T4   s_iclkrx0p9gh   || USBCLKM/P
AF1   AG1   s_iclkrx0p9gh   || CORECLKN/P
AM2   AN3   s_iclkrx0p9gh   || NETCPCLKN/P
|********************  MODEL SELECTORS ***************************
|---------------- DDR CLK_OUT IBIS Model -------------------
[Model Selector]   CLK_OUT
|pddrio.ibs   [18 October 2013 revision 0.1]
|renamed PDDRIO_D3FP3_
| ----------- DDR3 CLK_OUT Output Model Selector -----------
PDDRIO_D3FP3_34   DDR3 D3F_PDDRIO cell  Z0=34-Ohm
PDDRIO_D3FP3_40   DDR3 D3F_PDDRIO cell  Z0=40-Ohm
PDDRIO_D3FP3_48   DDR3 D3F_PDDRIO cell  Z0=48-Ohm
| ---------- DDR3L CLK_OUT Output Model Selector -----------
PDDRIO_D3FP3L_34   DDR3L D3F_PDDRIO cell  Z0=34-Ohm
PDDRIO_D3FP3L_40   DDR3L D3F_PDDRIO cell  Z0=40-Ohm
PDDRIO_D3FP3L_48   DDR3L D3F_PDDRIO cell  Z0=48-Ohm
|---------------- DDR ACC_OUT IBIS Model -------------------
[Model Selector]   ACC_OUT
|pddrio.ibs   [18 October 2013 revision 0.1]
|renamed PDDRIO_D3FP3_
| ---------- DDR3 ACC_OUT Output Model Selector ------------
PDDRIO_D3FP3_34   DDR3 D3F_PDDRIO cell  Z0=34-Ohm
PDDRIO_D3FP3_40   DDR3 D3F_PDDRIO cell  Z0=40-Ohm
PDDRIO_D3FP3_48   DDR3 D3F_PDDRIO cell  Z0=48-Ohm
| --------- DDR3L ACC_OUT Output Model Selector ------------
PDDRIO_D3FP3L_34   DDR3L D3F_PDDRIO cell  Z0=34-Ohm
PDDRIO_D3FP3L_40   DDR3L D3F_PDDRIO cell  Z0=40-Ohm
PDDRIO_D3FP3L_48   DDR3L D3F_PDDRIO cell  Z0=48-Ohm
|---------------- DDR DM IBIS Model -------------------
[Model Selector]   DM
|pddrio.ibs   [18 October 2013 revision 0.1]
|renamed PDDRIO_D3FP3_
| ------------- DDR3 DM Output Model Selector --------------
PDDRIO_D3FP3_34   DDR3 D3F_PDDRIO cell  Z0=34-Ohm
PDDRIO_D3FP3_40   DDR3 D3F_PDDRIO cell  Z0=40-Ohm
PDDRIO_D3FP3_48   DDR3 D3F_PDDRIO cell  Z0=48-Ohm
| ------------ DDR3L DM Output Model Selector --------------
PDDRIO_D3FP3L_34   DDR3L D3F_PDDRIO cell  Z0=34-Ohm
PDDRIO_D3FP3L_40   DDR3L D3F_PDDRIO cell  Z0=40-Ohm
PDDRIO_D3FP3L_48   DDR3L D3F_PDDRIO cell  Z0=48-Ohm
| -------------- DDR3 DM Input Model Selector --------------
PDDRIO_D3FP3_ODT120   DDR3 D3F_PDDRIO cell 120-Ohm ODT Receiver
PDDRIO_D3FP3_ODT40   DDR3 D3F_PDDRIO cell 40-Ohm ODT Receiver
PDDRIO_D3FP3_ODT60   DDR3 D3F_PDDRIO cell 60-Ohm ODT Receiver
PDDRIO_D3FP3_ODTOFF   DDR3 D3F_PDDRIO cell ODT off Receiver
| ------------- DDR3L DM Input Model Selector --------------
PDDRIO_D3FP3L_ODT120   DDR3L D3F_PDDRIO cell 120-Ohm ODT Receiver
PDDRIO_D3FP3L_ODT40   DDR3L D3F_PDDRIO cell 40-Ohm ODT Receiver
PDDRIO_D3FP3L_ODT60   DDR3L D3F_PDDRIO cell 60-Ohm ODT Receiver
PDDRIO_D3FP3L_ODTOFF   DDR3L D3F_PDDRIO cell ODT off Receiver
|---------------- DDR DQ IBIS Model -------------------
[Model Selector]   DQ
|pddrio.ibs   [18 October 2013 revision 0.1]
|renamed PDDRIO_D3FP3_
| -------------- DDR3 DQ Output Model Selector --------------
PDDRIO_D3FP3_34   DDR3 D3F_PDDRIO cell  Z0=34-Ohm
PDDRIO_D3FP3_40   DDR3 D3F_PDDRIO cell  Z0=40-Ohm
PDDRIO_D3FP3_48   DDR3 D3F_PDDRIO cell  Z0=48-Ohm
| ------------- DDR3L DQ Output Model Selector --------------
PDDRIO_D3FP3L_34   DDR3L D3F_PDDRIO cell  Z0=34-Ohm
PDDRIO_D3FP3L_40   DDR3L D3F_PDDRIO cell  Z0=40-Ohm
PDDRIO_D3FP3L_48   DDR3L D3F_PDDRIO cell  Z0=48-Ohm
| --------------- DDR3 DQ Input Model Selector --------------
PDDRIO_D3FP3_ODT120   DDR3 D3F_PDDRIO cell 120-Ohm ODT Receiver
PDDRIO_D3FP3_ODT40   DDR3 D3F_PDDRIO cell 40-Ohm ODT Receiver
PDDRIO_D3FP3_ODT60   DDR3 D3F_PDDRIO cell 60-Ohm ODT Receiver
PDDRIO_D3FP3_ODTOFF   DDR3 D3F_PDDRIO cell ODT off Receiver
| -------------- DDR3L DQ Input Model Selector --------------
PDDRIO_D3FP3L_ODT120   DDR3L D3F_PDDRIO cell 120-Ohm ODT Receiver
PDDRIO_D3FP3L_ODT40   DDR3L D3F_PDDRIO cell 40-Ohm ODT Receiver
PDDRIO_D3FP3L_ODT60   DDR3L D3F_PDDRIO cell 60-Ohm ODT Receiver
PDDRIO_D3FP3L_ODTOFF   DDR3L D3F_PDDRIO cell ODT off Receiver
| ----------------- DDR DQS IBIS Model --------------------
[Model Selector]   DQS
|pdiff.ibs   [18 October 2013 revision 0.1]
|renamed PDIFF_D3FP3_
| -------------- DDR3 DQS Input Model Selector ------------
PDIFF_D3FF3_ODT120   DDR3 D3F_PDIFF cell 120-Ohm ODT Receiver
PDIFF_D3FF3_ODT40   DDR3 D3F_PDIFF cell 40-Ohm ODT Receiver
PDIFF_D3FF3_ODT60   DDR3 D3F_PDIFF cell 60-Ohm ODT Receiver
PDIFF_D3FF3_ODTOFF   DDR3 D3F_PDIFF cell ODT off Receiver
| -------------- DDR3L DQS Input Model Selector ------------
PDIFF_D3FF3L_ODT120   DDR3L D3F_PDIFF cell 120-Ohm ODT Receiver
PDIFF_D3FF3L_ODT40   DDR3L D3F_PDIFF cell 40-Ohm ODT Receiver
PDIFF_D3FF3L_ODT60   DDR3L D3F_PDIFF cell 60-Ohm ODT Receiver
PDIFF_D3FF3L_ODTOFF   DDR3L D3F_PDIFF cell ODT off Receiver
| -------------- DDR3 DQS Output Model Selector ------------
PDIFF_D3FF3_34   DDR3 D3F_PDIFF cell  Z0=34-Ohm
PDIFF_D3FF3_40   DDR3 D3F_PDIFF cell  Z0=40-Ohm
PDIFF_D3FF3_48   DDR3 D3F_PDIFF cell  Z0=48-Ohm
| -------------- DDR3L DQS Output Model Selector -----------
PDIFF_D3FF3L_34   DDR3L D3F_PDIFF cell  Z0=34-Ohm
PDIFF_D3FF3L_40   DDR3L D3F_PDIFF cell  Z0=40-Ohm
PDIFF_D3FF3L_48   DDR3L D3F_PDIFF cell  Z0=48-Ohm
|----------------  iclkrx0p9gh IBIS Model --------------
[Model Selector]   iclkrx0p9gh
|iclkrx0p9gh_encmint_0.ibs   [12Feb12 revision 2.0]
|iclkrx0p9gh_encmint_1.ibs   [12Feb12 revision 2.0]
iclkrx0p9gh_encmint_0   Ext. CommMode Used
| When set to zero external common mode used
iclkrx0p9gh_encmint_1   Int. CommMode Used
| When set to one internal common mode used
|----------------  iclkrx0p9gv IBIS Model ---------------
[Model Selector]   iclkrx0p9gv
|iclkrx0p9gv_encmint_0.ibs   [12Feb12 revision 2.0]
|iclkrx0p9gv_encmint_1.ibs   [12Feb12 revision 2.0]
iclkrx0p9gv_encmint_0   Ext. CommMode Used
| When set to zero external common mode used
iclkrx0p9gv_encmint_1   Int. CommMode Used
| When set to one internal common mode used
|----------------  s_iclkrx0p9gh IBIS Model ---------------
[Model Selector]  s_iclkrx0p9gh
s_iclkrx0p9gh_encmint_0   Ext. CommMode Used
s_iclkrx0p9gh_encmint_1   Int. CommMode Used
|----------------  s_iclkrx0p9gv IBIS Model ---------------
[Model Selector]  s_iclkrx0p9gv
s_iclkrx0p9gv_encmint_0   Ext. CommMode Used
s_iclkrx0p9gv_encmint_1   Int. CommMode Used
|--------bc181540edc50bghypbfbh IBIS Model -----------
[Model Selector]   bc181540h
|bc181540edc50bghypbfbh.ibs   [23Jan12 revision 1.0]
bc181540h_40CCLASS_1P8  Cell operated at 1.8(nom)
|40CCLASS_1P8; 40C:130MHZ@5PF CLASS IO MODE
bc181540h_WK_PD_ON_1P8  Cell operated at 1.8(nom)
|WK_PD_ON_1P8; INPUT MODE WITH WK_PD_ON
bc181540h_40ECLASS_1P8  Cell operated at 1.8(nom)
|40ECLASS_1P8; 40E:230MHZ@5PF CLASS IO MODE
bc181540h_WK_PU_ON_1P8  Cell operated at 1.8(nom)
|WK_PU_ON_1P8; INPUT MODE WITH WK_PU_ON
bc181540h_40DCLASS_1P8  Cell operated at 1.8(nom)
|40DCLASS_1P8; 40D:200MHZ@5PF CLASS IO MODE
bc181540h_50BCLASS_1P8  Cell operated at 1.8(nom)
|50BCLASS_1P8; 50B:100MHZ@5PF CLASS IO MODE
|------ bc181540edc50bghypbfbv IBIS Model --------
[Model Selector]   bc181540v
|bc181540edc50bghypbfbv.ibs  [23Jan12 revision 1.0]
|bc181540v_40CCLASS_1P5  Cell operated at 1.5(nom)
|40CCLASS_1P5; 40C:130MHZ@5PF CLASS IO MODE
|bc181540v_WK_PD_ON_1P5  Cell operated at 1.5(nom)
|WK_PD_ON_1P5; INPUT MODE WITH WK_PD_ON
|bc181540v_40ECLASS_1P5  Cell operated at 1.5(nom)
|40ECLASS_1P5; 40E:230MHZ@5PF CLASS IO MODE
|bc181540v_WK_PU_ON_1P5  Cell operated at 1.5(nom)
|WK_PU_ON_1P5; INPUT MODE WITH WK_PU_ON
|bc181540v_40DCLASS_1P5  Cell operated at 1.5(nom)
|40DCLASS_1P5; 40D:200MHZ@5PF CLASS IO MODE
|bc181540v_50BCLASS_1P5  Cell operated at 1.5(nom)
|50BCLASS_1P5; 50B:100MHZ@5PF CLASS IO MODE
bc181540v_40CCLASS_1P8  Cell operated at 1.8(nom)
|40CCLASS_1P8; 40C:130MHZ@5PF CLASS IO MODE
bc181540v_WK_PD_ON_1P8  Cell operated at 1.8(nom)
|WK_PD_ON_1P8; INPUT MODE WITH WK_PD_ON
bc181540v_40ECLASS_1P8  Cell operated at 1.8(nom)
|40ECLASS_1P8; 40E:230MHZ@5PF CLASS IO MODE
bc181540v_WK_PU_ON_1P8  Cell operated at 1.8(nom)
|WK_PU_ON_1P8; INPUT MODE WITH WK_PU_ON
bc181540v_40DCLASS_1P8  Cell operated at 1.8(nom)
|40DCLASS_1P8; 40D:200MHZ@5PF CLASS IO MODE
bc181540v_50BCLASS_1P8  Cell operated at 1.8(nom)
|50BCLASS_1P8; 50B:100MHZ@5PF CLASS IO MODE
|--------bi2c1815gfzhsh IBIS Model ----------
[Model Selector]   bi2c1815gfzhsh
|bi2c1815gfzhsh.ibs   [11Jan12 revision 1.0]
bi2c1815h_HS_SLAVE_MODE_1P8  Cell operated at 1.8(nom)
|HS_SLAVE_MODE_1P8; I2C HS SLAVE MODE
bi2c1815h_FAST_STD_1P8  Cell operated at 1.8(nom)
|FAST_STD_1P8; I2C FAST AND STD MODE
bi2c1815h_HS_MASTER_MODE_1P8  Cell operated at 1.8(nom)
|HS_MASTER_MODE_1P8; I2C HS MASTER MODE
|--------- bi2c1815gfzhsv IBIS Model ------------
[Model Selector] bi2c1815gfzhsv
|bi2c1815gfzhsv.ibs   [11Jan12 revision 1.0]
bi2c1815v_HS_SLAVE_MODE_1P8  Cell operated at 1.8(nom)
|HS_SLAVE_MODE_1P8; I2C HS SLAVE MODE
bi2c1815v_FAST_STD_1P8  Cell operated at 1.8(nom)
|FAST_STD_1P8; I2C FAST AND STD MODE
bi2c1815v_HS_MASTER_MODE_1P8  Cell operated at 1.8(nom)
|HS_MASTER_MODE_1P8; I2C HS MASTER MODE
|------- ic1815ghypbfbh IBIS Model ------------
[Model Selector] ic1815ghypbfbh
|ic1815ghypbfbh.ibs   [27Dec11 revision 1.0]
ic1815h_WK_PD_ON_1P8  Cell operated at 1.8(nom)
|WK_PD_ON_1P8; WK_PD_ON
ic1815h_WK_PU_ON_1P8  Cell operated at 1.8(nom)
|WK_PU_ON_1P8; WK_PU_ON
ic1815h_RX_MODE_1P8  Cell operated at 1.8(nom)
|RX_MODE_1P8
|---------------- ic1815ghypbfbv IBIS Model --------
[Model Selector] ic1815ghypbfbv
|ic1815ghypbfbv.ibs   [27Dec11 revision 1.0]
ic1815v_WK_PD_ON_1P8  Cell operated at 1.8(nom)
|WK_PD_ON_1P8; WK_PD_ON
ic1815v_WK_PU_ON_1P8  Cell operated at 1.8(nom)
|WK_PU_ON_1P8; WK_PU_ON
ic1815v_RX_MODE_1P8  Cell operated at 1.8(nom)
|RX_MODE_1P8
|---------------- olvds18gh IBIS Model -----------
[Model Selector] olvds18gh
|olvds18gh.ibs   [30Dec11 revision 1.0]
OLVDS18GH_SUBLVDS_MODE_3MA_100_1P8  Cell operated at 1.8(nom)
|SUBLVDS MODE :3MA OUTPUT CURRENT SETTING WITH 100 OHM INT. TERM.
OLVDS18GH_2MA_200_1P8  Cell operated at 1.8(nom)
|2MA OUTPUT CURRENT SETTING WITH 200 OHM INT. TERM.
OLVDS18GH_4MA_100_1P8  Cell operated at 1.8(nom)
|4MA OUTPUT CURRENT SETTING WITH 100 OHM INT. TERM.
OLVDS18GH_SUBLVDS_MODE_2.5MA_100_1P8  Cell operated at 1.8(nom)
|SUBLVDS MODE : 2.5MA OUTPUT CURRENT SETTING WITH 100 OHM INT. TERM.
OLVDS18GH_3.5MA_100_1P8  Cell operated at 1.8(nom)
|3.5MA OUTPUT CURRENT SETTING WITH 100 OHM INT. TERM.
OLVDS18GH_SUBLVDS_MODE_2.66MA_200_1P8  Cell operated at 1.8(nom)
|SUBLVDS MODE :2.66MA OUTPUT CURRENT SETTING WITH 200 OHM INT. TERM.
OLVDS18GH_SUBLVDS_MODE_2MA_200_1P8  Cell operated at 1.8(nom)
|SUBLVDS MODE :2MA OUTPUT CURRENT SETTING WITH 200 OHM INT. TERM.
OLVDS18GH_4MA_200_1P8  Cell operated at 1.8(nom)
|4MA OUTPUT CURRENT SETTING WITH 200 OHM INT. TERM.
OLVDS18GH_3.33MA_200_1P8  Cell operated at 1.8(nom)
|3.33MA OUTPUT CURRENT SETTING WITH 200 OHM INT. TERM.
OLVDS18GH_SUBLVDS_MODE_4MA_100_1P8  Cell operated at 1.8(nom)
|SUBLVDS MODE :4MA OUTPUT CURRENT SETTING WITH 100 OHM INT. TERM.
OLVDS18GH_SUBLVDS_MODE_3.5MA_100_1P8  Cell operated at 1.8(nom)
|SUBLVDS MODE :3.5MA OUTPUT CURRENT SETTING WITH 100 OHM INT. TERM.
OLVDS18GH_3MA_100_1P8  Cell operated at 1.8(nom)
|3MA OUTPUT CURRENT SETTING WITH 100 OHM INT. TERM.
OLVDS18GH_SUBLVDS_MODE_4MA_200_1P8  Cell operated at 1.8(nom)
|SUBLVDS MODE :4MA OUTPUT CURRENT SETTING WITH 200 OHM INT. TERM.
OLVDS18GH_2.5MA_100_1P8  Cell operated at 1.8(nom)
|2.5MA OUTPUT CURRENT SETTING WITH 100 OHM INT. TERM.
OLVDS18GH_SUBLVDS_MODE_3.33MA_200_1P8  Cell operated at 1.8(nom)
|SUBLVDS MODE :3.33MA OUTPUT CURRENT SETTING WITH 200 OHM INT. TERM.
OLVDS18GH_2.66MA_200_1P8  Cell operated at 1.8(nom)
|   Package Model Definition
[Define Package Model]  66ak2eXX
[Manufacturer]   Texas Instruments Incorporated
[OEM]   Texas Instruments Incorporated
[Description]   66ak2eXX pkg with all signals except AMI
|   file: pgr6990a-e5_100313
[Number Of Pins]   470
[Pin Numbers]
AF31 | 1   BGA-AF31 BOOTCOMPLETE
AG32 | 2   BGA-AG32 TRST
AH33 | 3   BGA-AH33 POR
AF32 | 4   BGA-AF32 RESETFULL
AG31 | 5   BGA-AG31 TDI
AG30 | 6   BGA-AG30 SCL0
AF30 | 7   BGA-AF30 HOUT
AE30 | 8   BGA-AE30 RSV030
AD32 | 9   BGA-AD32 GPIO27
AD33 | 10  BGA-AD33 GPIO28
AD30 | 11  BGA-AD30 GPIO31
AH30 | 12  BGA-AH30 SCL1
AD31 | 13  BGA-AD31 GPIO29
AH32 | 14  BGA-AH32 TMS
AE33 | 15  BGA-AE33 GPIO30
AG33 | 16  BGA-AG33 RSV028
AJ33 | 17  BGA-AJ33 TCK
AH29 | 18  BGA-AH29 RESETSTAT
AH31 | 19  BGA-AH31 SCL2
AE29 | 20  BGA-AE29 RESET
AF29 | 21  BGA-AF29 TDO
AF33 | 22  BGA-AF33 RSV029
AG29 | 23  BGA-AG29 SDA2
AC31 | 24  BGA-AC31 GPIO23
AJ32 | 25  BGA-AJ32 SDA1
AC30 | 26  BGA-AC30 GPIO26
AC32 | 27  BGA-AC32 GPIO24
AK33 | 28  BGA-AK33 TSIP0CLKB
AC33 | 29  BGA-AC33 GPIO21
AJ31 | 30  BGA-AJ31 TSIP0FSA
AG28 | 31  BGA-AG28 SDA0
AD29 | 32  BGA-AD29 GPIO22
AB30 | 33  BGA-AB30 GPIO25
AK32 | 34  BGA-AK32 TSIP0FSB
AM31 | 35  BGA-AM31 TSIP0TR0
AK29 | 36  BGA-AK29 SGMII0TXN1
AL33 | 37  BGA-AL33 TSIP0TR1
AJ28 | 38  BGA-AJ28 RSV018
AC29 | 39  BGA-AC29 GPIO20
AB32 | 40  BGA-AB32 GPIO17
AL32 | 41  BGA-AL32 TSIP0TX0
AB31 | 42  BGA-AB31 GPIO19
AJ27 | 43  BGA-AJ27 SGMII00REFRES
AB33 | 44  BGA-AB33 GPIO18
AB29 | 45  BGA-AB29 GPIO10
AL30 | 46  BGA-AL30 SGMII0TXN0
AN30 | 47  BGA-AN30 SGMII0RXP0
AK28 | 48  BGA-AK28 SGMII0TXP1
AA33 | 49  BGA-AA33 GPIO16
AM32 | 50  BGA-AM32 TSIP0TX1
AN29 | 51  BGA-AN29 SGMII0RXN0
AK31 | 52  BGA-AK31 TSIP0CLKA
AJ26 | 53  BGA-AJ26 RSV019
AA30 | 54  BGA-AA30 GPIO13
AL29 | 55  BGA-AL29 SGMII0TXP0
AA29 | 56  BGA-AA29 GPIO01
AL26 | 57  BGA-AL26 SGMII0TXP2
AM29 | 58  BGA-AM29 SGMII0RXP1
Y33  | 59  BGA-Y33 GPIO14
Y29  | 60  BGA-Y29 GPIO02
Y32  | 61  BGA-Y32 GPIO12
AJ22 | 62  BGA-AJ22 SGMII01REFRES
AJ25 | 63  BGA-AJ25 SGMII0CLKN
AM28 | 64  BGA-AM28 SGMII0RXN1
AL27 | 65  BGA-AL27 SGMII0TXN2
Y30  | 66  BGA-Y30 GPIO11
Y31  | 67  BGA-Y31 GPIO15
AN27 | 68  BGA-AN27 SGMII0RXP2
W33  | 69  BGA-W33 GPIO09
W29  | 70  BGA-W29 UART0DSR
W32  | 71  BGA-W32 GPIO06
AJ20 | 72  BGA-AJ20 RSV016
AM26 | 73  BGA-AM26 SGMII0RXP3
AN26 | 74  BGA-AN26 SGMII0RXN2
AK26 | 75  BGA-AK26 SGMII0TXN3
AJ24 | 76  BGA-AJ24 SGMII0CLKP
W31  | 77  BGA-W31 GPIO08
AM25 | 78  BGA-AM25 SGMII0RXN3
V33  | 79  BGA-V33 GPIO03
U29  | 80  BGA-U29 UART1RXD
W30  | 81  BGA-W30 GPIO05
AK25 | 82  BGA-AK25 SGMII0TXP3
AN24 | 83  BGA-AN24 SGMII0RXP4
V32  | 84  BGA-V32 GPIO04
V31  | 85  BGA-V31 GPIO07
T29  | 86  BGA-T29 UART0RXD
AL24 | 87  BGA-AL24 SGMII0TXN4
V30  | 88  BGA-V30 GPIO00
V29  | 89  BGA-V29 VCL
AN23 | 90  BGA-AN23 SGMII0RXN4
U30  | 91  BGA-U30 VD
U33  | 92  BGA-U33 UART0DTR
AK23 | 93  BGA-AK23 SGMII0TXN5
AL23 | 94  BGA-AL23 SGMII0TXP4
R30  | 95  BGA-R30 SPI1DIN
AM23 | 96  BGA-AM23 SGMII0RXP5
T33  | 97  BGA-T33 UART1RTS
R29  | 98  BGA-R29 SPI2SCS1
T32  | 99  BGA-T32 UART1TXD
AG14 | 100 BGA-AG14 PCIE0REFRES
AM22 | 101 BGA-AM22 SGMII0RXN5
T31  | 102 BGA-T31 UART1CTS
P30  | 103 BGA-P30 SPI2DIN
R33  | 104 BGA-R33 UART0CTS
T30  | 105 BGA-T30 UART0TXD
AK22 | 106 BGA-AK22 SGMII0TXP5
R32  | 107 BGA-R32 UART0RTS
P29  | 108 BGA-P29 SPI1SCS0
AN21 | 109 BGA-AN21 SGMII0RXP6
P33  | 110 BGA-P33 SPI2SCS2
AN20 | 111 BGA-AN20 SGMII0RXN6
R31  | 112 BGA-R31 SPI2DOUT
K32  | 113 BGA-K32 TIMI1
AK20 | 114 BGA-AK20 SGMII0TXN7
AL21 | 115 BGA-AL21 SGMII0TXN6
P32  | 116 BGA-P32 SPI1DOUT
N33  | 117 BGA-N33 SPI1SCS3
AG12 | 118 BGA-AG12 RSV017
P31  | 119 BGA-P31 SPI2SCS0
AL20 | 120 BGA-AL20 SGMII0TXP6
AM20 | 121 BGA-AM20 SGMII0RXP7
M33  | 122 BGA-M33 SPI1CLK
L29  | 123 BGA-L29 SPI0SCS2
AM19 | 124 BGA-AM19 SGMII0RXN7
N30  | 125 BGA-N30 SPI1SCS2
AJ10 | 126 BGA-AJ10 PCIE1REFRES
M32  | 127 BGA-M32 SPI1SCS1
AK19 | 128 BGA-AK19 SGMII0TXP7
N29  | 129 BGA-N29 SPI0DOUT
M31  | 130 BGA-M31 SPI0DIN
M29  | 131 BGA-M29 SPI0SCS1
L31  | 132 BGA-L31 SPI0SCS0
M30  | 133 BGA-M30 SPI0CLK
L33  | 134 BGA-L33 SPI2CLK
K31  | 135 BGA-K31 TIMO0
L32  | 136 BGA-L32 SPI0SCS3
L30  | 137 BGA-L30 SPI2SCS3
K33  | 138 BGA-K33 TIMI0
K29  | 139 BGA-K29 USIMRST
J33  | 140 BGA-J33 USIMCLK
K30  | 141 BGA-K30 TIMO1
H33  | 142 BGA-H33 USIMIO
J32  | 143 BGA-J32 RSV001
H32  | 144 BGA-H32 RSV000
AJ18 | 145 BGA-AJ18 PCIE0CLKN
J30  | 146 BGA-J30 RSV013
J29  | 147 BGA-J29 RSV014
AL18 | 148 BGA-AL18 PCIE0TXN0
AJ17 | 149 BGA-AJ17 PCIE0CLKP
AK17 | 150 BGA-AK17 PCIE0TXN1
AN18 | 151 BGA-AN18 PCIE0RXP0
AL17 | 152 BGA-AL17 PCIE0TXP0
AM17 | 153 BGA-AM17 PCIE0RXP1
AK16 | 154 BGA-AK16 PCIE0TXP1
AN17 | 155 BGA-AN17 PCIE0RXN0
AM16 | 156 BGA-AM16 PCIE0RXN1
AJ15 | 157 BGA-AJ15 PCIE1CLKN
AL15 | 158 BGA-AL15 PCIE1TXN0
AN15 | 159 BGA-AN15 PCIE1RXP0
AL14 | 160 BGA-AL14 PCIE1TXP0
AN14 | 161 BGA-AN14 PCIE1RXN0
AJ14 | 162 BGA-AJ14 PCIE1CLKP
AK14 | 163 BGA-AK14 PCIE1TXN1
AM14 | 164 BGA-AM14 PCIE1RXP1
AK13 | 165 BGA-AK13 PCIE1TXP1
AM13 | 166 BGA-AM13 PCIE1RXN1
AL12 | 167 BGA-AL12 XFITXN0
AN12 | 168 BGA-AN12 XFIRXP0
AL11 | 169 BGA-AL11 XFITXP0
AN11 | 170 BGA-AN11 XFIRXN0
AG10 | 171 BGA-AG10 XFIREFRES0
AJ11 | 172 BGA-AJ11 XFICLKP
AJ12 | 173 BGA-AJ12 XFICLKN
AH9  | 174 BGA-AH9 RSV020
AH7  | 175 BGA-AH7 XFIREFRES1
AK11 | 176 BGA-AK11 XFITXN1
AM11 | 177 BGA-AM11 XFIRXP1
F33  | 178 BGA-F33 DDRD57
AK10 | 179 BGA-AK10 XFITXP1
C33  | 180 BGA-C33 DDRDQS7P
AM10 | 181 BGA-AM10 XFIRXN1
D33  | 182 BGA-D33 DDRDQS7N
E33  | 183 BGA-E33 DDRD60
AL9  | 184 BGA-AL9 HYPLNK0TXN0
B32  | 185 BGA-B32 DDRD63
AN9  | 186 BGA-AN9 HYPLNK0RXP0
F32  | 187 BGA-F32 DDRD58
E31  | 188 BGA-E31 DDRDQM6
AL8  | 189 BGA-AL8 HYPLNK0TXP0
C30  | 190 BGA-C30 DDRD53
AN8  | 191 BGA-AN8 HYPLNK0RXN0
F31  | 192 BGA-F31 DDRD56
E32  | 193 BGA-E32 DDRD59
AK8  | 194 BGA-AK8 HYPLNK0TXN1
C32  | 195 BGA-C32 DDRD61
A30  | 196 BGA-A30 DDRDQS6P
B31  | 197 BGA-B31 DDRD50
AM8  | 198 BGA-AM8 HYPLNK0RXP1
B30  | 199 BGA-B30 DDRDQS6N
AK7  | 200 BGA-AK7 HYPLNK0TXP1
D30  | 201 BGA-D30 DDRD55
A29  | 202 BGA-A29 DDRD48
D32  | 203 BGA-D32 DDRD62
AM7  | 204 BGA-AM7 HYPLNK0RXN1
D28  | 205 BGA-D28 DDRD41
G18  | 206 BGA-G18 DDRRZQ2
AJ7  | 207 BGA-AJ7 HYPLNK0CLKP
B29  | 208 BGA-B29 DDRD52
A31  | 209 BGA-A31 DDRDQM7
AJ8  | 210 BGA-AJ8 HYPLNK0CLKN
B28  | 211 BGA-B28 DDRD44
AG8  | 212 BGA-AG8 RSV015
E30  | 213 BGA-E30 DDRD54
AJ5  | 214 BGA-AJ5 HYPLNK0REFRES
AL6  | 215 BGA-AL6 HYPLNK0TXN2
AN6  | 216 BGA-AN6 HYPLNK0RXP2
C26  | 217 BGA-C26 DDRD47
E29  | 218 BGA-E29 DDRD51
E26  | 219 BGA-E26 DDRDQM4
AL5  | 220 BGA-AL5 HYPLNK0TXP2
C28  | 221 BGA-C28 DDRD42
A28  | 222 BGA-A28 DDRD49
A27  | 223 BGA-A27 DDRDQS5P
AN5  | 224 BGA-AN5 HYPLNK0RXN2
E28  | 225 BGA-E28 DDRD40
E25  | 226 BGA-E25 DDRD37
B27  | 227 BGA-B27 DDRDQS5N
AK5  | 228 BGA-AK5 HYPLNK0TXN3
A26  | 229 BGA-A26 DDRD45
E27  | 230 BGA-E27 DDRD43
AM5  | 231 BGA-AM5 HYPLNK0RXP3
D24  | 232 BGA-D24 DDRD34
B23  | 233 BGA-B23 DDRD32
AK4  | 234 BGA-AK4 HYPLNK0TXP3
AF6  | 235 BGA-AF6 XFIMDCLK
A25  | 236 BGA-A25 DDRD39
AM4  | 237 BGA-AM4 HYPLNK0RXN3
B26  | 238 BGA-B26 DDRD46
A24  | 239 BGA-A24 DDRDQS4P
D26  | 240 BGA-D26 DDRDQM5
AJ1  | 241 BGA-AJ1 TSRXCLKOUT0P
E22  | 242 BGA-E22 DDRCB02
AL1  | 243 BGA-AL1 TSPUSHEVT1
C22  | 244 BGA-C22 DDRCB04
AH6  | 245 BGA-AH6 MDCLK0
AJ3  | 246 BGA-AJ3 HYPLNK0RXFLCLK
AK2  | 247 BGA-AK2 TSREFCLKP
AF1  | 248 BGA-AF1 CORECLKP
E24  | 249 BGA-E24 DDRD36
AG2  | 250 BGA-AG2 TSRXCLKOUT1P
B25  | 251 BGA-B25 DDRD38
AL3  | 252 BGA-AL3 RSV006
B24  | 253 BGA-B24 DDRDQS4N
AH5  | 254 BGA-AH5 MDIO0
AN3  | 255 BGA-AN3 NETCPCLKN
AJ2  | 256 BGA-AJ2 TSRXCLKOUT0N
B22  | 257 BGA-B22 DDRDQS8P
AE2  | 258 BGA-AE2 RSV002
AG6  | 259 BGA-AG6 NETCPCLKSEL
AE5  | 260 BGA-AE5 TSSYNCEVT
A21  | 261 BGA-A21 DDRCB07
AK1  | 262 BGA-AK1 TSREFCLKN
AG1  | 263 BGA-AG1 CORECLKN
A22  | 264 BGA-A22 DDRDQS8N
A23  | 265 BGA-A23 DDRCB00
C24  | 266 BGA-C24 DDRD35
AH1  | 267 BGA-AH1 TSRXCLKOUT1N
AB6  | 268 BGA-AB6 HYPLNK0TXPMCLK
AL2  | 269 BGA-AL2 RSV007
E23  | 270 BGA-E23 DDRD33
AF4  | 271 BGA-AF4 TSCOMPOUT
AC6  | 272 BGA-AC6 HYPLNK0TXFLCLK
AM2  | 273 BGA-AM2 NETCPCLKP
AF2  | 274 BGA-AF2 RSV003
AE7  | 275 BGA-AE7 XFIMDIO
AC5  | 276 BGA-AC5 EMU00
B18  | 277 BGA-B18 DDRBA2
AH4  | 278 BGA-AH4 HYPLNK0TXFLDAT
D20  | 279 BGA-D20 DDRRESET
AH2  | 280 BGA-AH2 EMU18
D22  | 281 BGA-D22 DDRCB01
AD6  | 282 BGA-AD6 EMU04
AE1  | 283 BGA-AE1 HYPLNK0RXPMCLK
AE4  | 284 BGA-AE4 SYSCLKOUT
E21  | 285 BGA-E21 DDRCB03
AG3  | 286 BGA-AG3 TSPUSHEVT0
AB4  | 287 BGA-AB4 EMU08
AE6  | 288 BGA-AE6 EMU03
AE3  | 289 BGA-AE3 HYPLNK0RXFLDAT
E20  | 290 BGA-E20 RSV022
B21  | 291 BGA-B21 DDRCB05
B17  | 292 BGA-B17 DDRA09
W3   | 293 BGA-W3 USB0DM
AG4  | 294 BGA-AG4 EMU11
AD3  | 295 BGA-AD3 EMU05
E19  | 296 BGA-E19 DDRA15
AA6  | 297 BGA-AA6 EMU01
AG5  | 298 BGA-AG5 RSV008
W4   | 299 BGA-W4 USB0ID0
AA5  | 300 BGA-AA5 EMU15
AH3  | 301 BGA-AH3 EMU09
AC4  | 302 BGA-AC4 EMU02
Y2   | 303 BGA-Y2 EMIFOE
AD1  | 304 BGA-AD1 HYPLNK0RXPMDAT
A20  | 305 BGA-A20 DDRCB06
C20  | 306 BGA-C20 DDRCKE0
AC2  | 307 BGA-AC2 EMU13
W8   | 308 BGA-W8 RSV011
AC3  | 309 BGA-AC3 EMU07
AF5  | 310 BGA-AF5 HYPLNK0TXPMDAT
V3   | 311 BGA-V3 USB0DP
D18  | 312 BGA-D18 DDRA11
AD2  | 313 BGA-AD2 EMU12
AA2  | 314 BGA-AA2 EMIFBE0
AB5  | 315 BGA-AB5 EMU06
A19  | 316 BGA-A19 DDRCKE1
W5   | 317 BGA-W5 USB0VBUS
B20  | 318 BGA-B20 DDRDQM8
E18  | 319 BGA-E18 DDRA12
AB2  | 320 BGA-AB2 EMU16
AC1  | 321 BGA-AC1 USB1DRVVBUS
AF3  | 322 BGA-AF3 EMU10
C16  | 323 BGA-C16 DDRA03
W1   | 324 BGA-W1 EMIFCE2
B19  | 325 BGA-B19 RSV021
D15  | 326 BGA-D15 DDRA00
AB3  | 327 BGA-AB3 EMU14
W7   | 328 BGA-W7 RSV012
Y4   | 329 BGA-Y4 EMIFCE1
D16  | 330 BGA-D16 DDRA04
Y5   | 331 BGA-Y5 EMU17
AA1  | 332 BGA-AA1 EMIFCE0
A18  | 333 BGA-A18 DDRA08
C18  | 334 BGA-C18 DDRA14
AB1  | 335 BGA-AB1 USB0DRVVBUS
Y1   | 336 BGA-Y1 EMIFCE3
V2   | 337 BGA-V2 USB0TX0P
E17  | 338 BGA-E17 DDRA07
Y6   | 339 BGA-Y6 USB0RESREF
Y3   | 340 BGA-Y3 EMIFRNW
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| Models and submodels in the file (103): PDDRIO_D3FP3_34 (I/O), PDDRIO_D3FP3_40 (I/O), PDDRIO_D3FP3_48 (I/O), PDDRIO_D3FP3_ODT120 (Input), PDDRIO_D3FP3_ODT40 (Input), PDDRIO_D3FP3_ODT60 (Input), PDDRIO_D3FP3_ODTOFF (Input), PDDRIO_D3FP3L_34 (I/O), PDDRIO_D3FP3L_40 (I/O), PDDRIO_D3FP3L_48 (I/O), PDDRIO_D3FP3L_ODT120 (Input), PDDRIO_D3FP3L_ODT40 (Input), PDDRIO_D3FP3L_ODT60 (Input), PDDRIO_D3FP3L_ODTOFF (Input), PDIFF_D3FF3_34 (I/O), PDIFF_D3FF3_40 (I/O), PDIFF_D3FF3_48 (I/O), PDIFF_D3FF3_ODT120 (Input), PDIFF_D3FF3_ODT40 (Input), PDIFF_D3FF3_ODT60 (Input), PDIFF_D3FF3_ODTOFF (Input), PDIFF_D3FF3L_34 (I/O), PDIFF_D3FF3L_40 (I/O), PDIFF_D3FF3L_48 (I/O), PDIFF_D3FF3L_ODT120 (Input), PDIFF_D3FF3L_ODT40 (Input), PDIFF_D3FF3L_ODT60 (Input), PDIFF_D3FF3L_ODTOFF (Input), bc181540h_40CCLASS_1P5 (I/O), bc181540h_WK_PD_ON_1P5 (Input), bc181540h_40ECLASS_1P5 (I/O), bc181540h_WK_PU_ON_1P5 (Input), bc181540h_40DCLASS_1P5 (I/O), bc181540h_50BCLASS_1P5 (I/O), bc181540h_40CCLASS_1P8 (I/O), bc181540h_WK_PD_ON_1P8 (Input), bc181540h_40ECLASS_1P8 (I/O), bc181540h_WK_PU_ON_1P8 (Input), bc181540h_40DCLASS_1P8 (I/O), bc181540h_50BCLASS_1P8 (I/O), bc181540v_40CCLASS_1P5 (I/O), bc181540v_WK_PD_ON_1P5 (Input), bc181540v_40ECLASS_1P5 (I/O), bc181540v_WK_PU_ON_1P5 (Input), bc181540v_40DCLASS_1P5 (I/O), bc181540v_50BCLASS_1P5 (I/O), bc181540v_40CCLASS_1P8 (I/O), bc181540v_WK_PD_ON_1P8 (Input), bc181540v_40ECLASS_1P8 (I/O), bc181540v_WK_PU_ON_1P8 (Input), bc181540v_40DCLASS_1P8 (I/O), bc181540v_50BCLASS_1P8 (I/O), bi2c1815h_HS_SLAVE_MODE_1P5 (I/O_open_drain), bi2c1815h_FAST_STD_1P5 (I/O_open_drain), bi2c1815h_HS_MASTER_MODE_1P5 (I/O), bi2c1815h_HS_SLAVE_MODE_1P8 (I/O_open_drain), bi2c1815h_FAST_STD_1P8 (I/O_open_drain), bi2c1815h_HS_MASTER_MODE_1P8 (I/O), bi2c1815v_HS_SLAVE_MODE_1P5 (I/O_open_drain), bi2c1815v_FAST_STD_1P5 (I/O_open_drain), bi2c1815v_HS_MASTER_MODE_1P5 (I/O), bi2c1815v_HS_SLAVE_MODE_1P8 (I/O_open_drain), bi2c1815v_FAST_STD_1P8 (I/O_open_drain), bi2c1815v_HS_MASTER_MODE_1P8 (I/O), ic1815h_WK_PD_ON_1P5 (Input), ic1815h_WK_PU_ON_1P5 (Input), ic1815h_RX_MODE_1P5 (Input), ic1815h_WK_PD_ON_1P8 (Input), ic1815h_WK_PU_ON_1P8 (Input), ic1815h_RX_MODE_1P8 (Input), ic1815v_WK_PD_ON_1P5 (Input), ic1815v_WK_PU_ON_1P5 (Input), ic1815v_RX_MODE_1P5 (Input), ic1815v_WK_PD_ON_1P8 (Input), ic1815v_WK_PU_ON_1P8 (Input), ic1815v_RX_MODE_1P8 (Input), iclkrx0p9gh_encmint_0 (Input), s_iclkrx0p9gh_encmint_0 (Series), iclkrx0p9gh_encmint_1 (Input), s_iclkrx0p9gh_encmint_1 (Series)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
